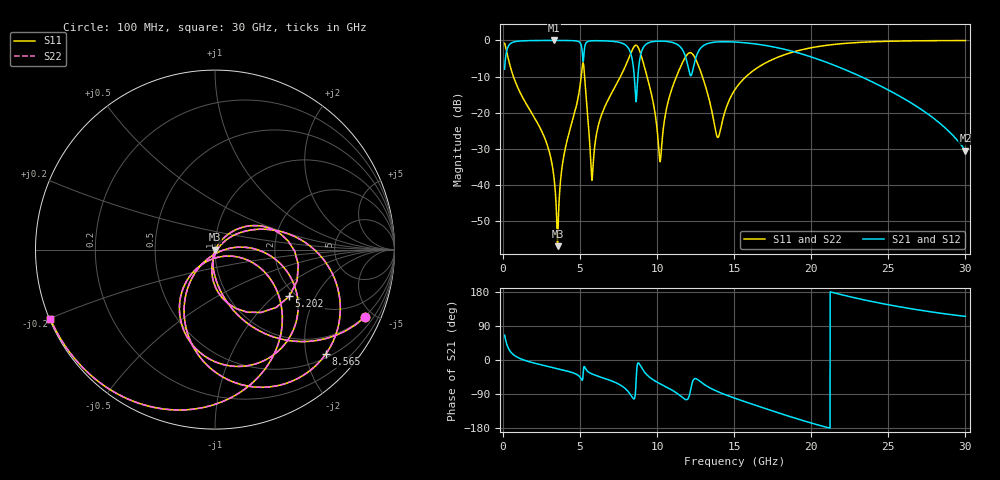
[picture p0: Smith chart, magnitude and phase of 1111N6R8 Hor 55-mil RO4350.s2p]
# GHz S MA R 50
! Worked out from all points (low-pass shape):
!   3201 points, 100 MHz to 30 GHz, reference 50 ohm
!   highest |S21| = -0.01 dB at 3.305 GHz (marker M1); lowest = -30.5 dB at 30 GHz (marker M2)
!   |S21| within 3 dB of the highest: 228 MHz to 5.134 GHz (4.906 GHz wide, 183 % of centre); 12.68 GHz to 18.78 GHz (6.097 GHz wide, 38.8 % of centre)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
!   lowest |S11| = -56.9 dB at 3.538 GHz (marker M3), VSWR 1.00, Z = 50.1 - j0.0335 ohm
!   |S11| at or under -10 dB: 670.4 MHz to 5.069 GHz (4.399 GHz wide, 153 % of centre); 5.291 GHz to 7.615 GHz (2.324 GHz wide, 36 % of centre); 12.93 GHz to 15.77 GHz (2.833 GHz wide, 19.7 % of centre)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
!   |S22| runs from -56.9 to 0.0 dB; largest |S21 - S12| = 0
!   S11 on the Smith chart (normalised r, x): 100 MHz: 0.95, -4.45; 5.202 GHz: 1.85, -1.27; 8.565 GHz: 0.57, -2.39; 30 GHz: 0.00, -0.20
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0.1  0.916 -24.3  0.4009 65.7  0.4009 65.7  0.916 -24.3
0.7634062  0.2792 -78.7  0.9596 11.2  0.9596 11.2  0.2792 -78.7
2.71625  0.04392 -103.7  0.9977 -15.1  0.9977 -15.1  0.04392 -103.7
3.304906  0.0127 -104.9  0.9983 -20.6  0.9983 -20.6  0.0127 -104.9
3.5385  0.001433 -13.5  0.9982 -22.8  0.9982 -22.8  0.001433 -13.5
3.949625  0.02589 58.9  0.9973 -26.9  0.9973 -26.9  0.02589 58.9
5.089563  0.3463 18.4  0.8261 -51.5  0.8261 -51.5  0.3463 18.4
5.201688  0.4888 -32.2  0.5108 -34.2  0.5108 -34.2  0.4888 -32.2
5.799688  0.01347 -0.1  0.9886 -37.3  0.9886 -37.3  0.01347 -0.1
6.350969  0.08849 40.5  0.9889 -45.3  0.9889 -45.3  0.08849 40.5
7.892688  0.4193 12.0  0.8791 -74.2  0.8791 -74.2  0.4193 12.0
8.565437  0.8487 -43.4  0.2193 -95.3  0.2193 -95.3  0.8487 -43.4
9.088688  0.4986 -107.5  0.7885 -26.9  0.7885 -26.9  0.4986 -107.5
10.06978  0.03941 -117.3  0.977 -60.1  0.977 -60.1  0.03941 -117.3
11.26578  0.323 -7.5  0.8892 -87.2  0.8892 -87.2  0.323 -7.5
12.03197  0.6635 -56.8  0.405 -99.8  0.405 -99.8  0.6635 -56.8
12.68603  0.4432 -115.4  0.7106 -53.4  0.7106 -53.4  0.4432 -115.4
13.91006  0.0458 -81.5  0.9527 -83.1  0.9527 -83.1  0.0458 -81.5
15.05  0.2091 -18.5  0.9492 -101.0  0.9492 -101.0  0.2091 -18.5
20.03956  0.7948 -78.0  0.587 -166.8  0.587 -166.8  0.7948 -78.0
25.01978  0.9726 -125.3  0.2052 145.7  0.2052 145.7  0.9726 -125.3
30  0.9952 -157.1  0.02984 115.2  0.02984 115.2  0.9952 -157.1
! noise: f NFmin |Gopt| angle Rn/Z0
0.1  0.001241  0.853  2.37  0.0018
3.417  0.009563  0.4702  22.17  0.002957
6.743  0.02917  0.6294  41.7  0.01299
10.06  0.06132  0.7279  62.03  0.03322
13.39  0.1306  0.8244  80.37  0.09178
16.7  0.08078  0.6814  95.3  0.02324
20.03  0.09963  0.7048  108.9  0.02374
23.35  0.154  0.791  123.8  0.03529
26.67  0.3088  0.8912  140.6  0.07216
30  1.202  0.9714  157.6  0.3661
